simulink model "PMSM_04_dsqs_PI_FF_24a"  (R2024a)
settings: Solver=ode45  StartTime=0.0  StopTime=0.1  MaxStep=1e-4  RelTol=1e-3  AbsTol=1e-4  EnableMultiTasking=on
undefined symbols (not defined in the file): by, established, Flux, linkage, magnets, V
libraries: spsControlledVoltageSourceLib x3, spsCurrentMeasurementLib x3, slpidlib x2, spsPermanentMagnetSynchronousMachineLib x1, spspowerguiLib x1

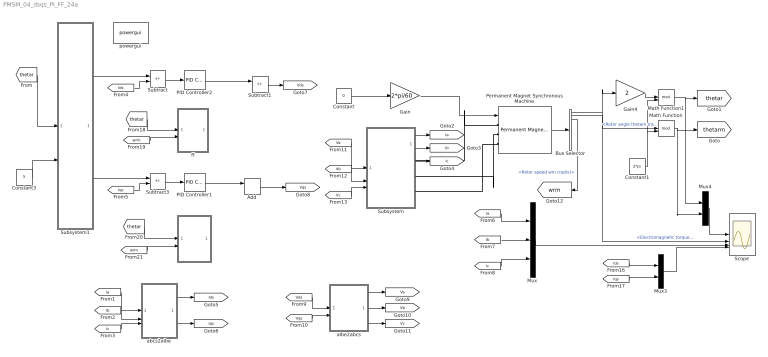
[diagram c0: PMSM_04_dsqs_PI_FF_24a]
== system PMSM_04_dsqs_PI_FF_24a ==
  Add : Sum
  Bus Selector : BusSelector  OutputSignals=Rotor angle thetam (rad),Electromagnetic torque Te (N*m),Rotor speed wm (rad/s)
  Constant : Constant  Value=0
  Constant1 : Constant  Value=2*pi
  Constant3 : Constant  Value=3
  FF : Subsystem
  Gain : Gain  Gain=2*pi/60
  Gain4 : Gain  Gain=2
  Math Function : Math  Operator=mod  SignedPower=on
  Math Function1 : Math  Operator=mod  SignedPower=on
  Mux : Mux  Inputs=3
  Mux3 : Mux  Inputs=2
  Mux4 : Mux  Inputs=2
  PID Controller1 : slpidlib/PID Controller  Controller=PI  Form=Parallel  TimeDomain=Continuous-time  UseExternalTs=off  SampleTime=1  IntegratorMethod=Forward Euler  FilterMethod=Forward Euler  ControllerParametersSource=internal  P=2*pi*500*0.00476  I=2*pi*500*0.423  UseKiTs=off  D=0  UseExternalDerivativeSource=off  N=100  UseFilter=on  TunerSelectOption=Transfer Function Based (PID Tuner App)  InitialConditionSource=internal  InitialConditionForIntegrator=0  InitialConditionForFilter=0  DifferentiatorICPrevScaledInput=0  ExternalReset=none  TrackingMode=off  Kt=1  LimitOutput=off  SatLimitsSource=internal  UpperSaturationLimit=inf  LowerSaturationLimit=-inf  LinearizeAsGain=on  AntiWindupMode=none  Kb=1  LimitIntegrator=off  UpperIntegratorSaturationLimit=inf  LowerIntegratorSaturationLimit=-inf  POutMin=[]  POutMax=[]  IOutMin=[]  IOutMax=[]  DOutMin=[]  DOutMax=[]  NOutMin=[]  NOutMax=[]  SumOutMin=[]  SumOutMax=[]  SaturationOutMin=[]  SaturationOutMax=[]  PParamMin=[]  PParamMax=[]  IParamMin=[]  IParamMax=[]  DParamMin=[]  DParamMax=[]  NParamMin=[]  NParamMax=[]  KbParamMin=[]  KbParamMax=[]  KtParamMin=[]  KtParamMax=[]  KbOutMin=[]  KbOutMax=[]  KtOutMin=[]  KtOutMax=[]  IntegratorOutMin=[]  IntegratorOutMax=[]  FilterOutMin=[]  FilterOutMax=[]  SumI1OutMin=[]  SumI1OutMax=[]  SumI2OutMin=[]  SumI2OutMax=[]  SumI3OutMin=[]  SumI3OutMax=[]  SumI4OutMin=[]  SumI4OutMax=[]  SumDOutMin=[]  SumDOutMax=[]  DifferentiatorOutMin=[]  DifferentiatorOutMax=[]  FilterDiffOutCoefMin=[]  FilterDiffOutCoefMax=[]  ReciprocalOutMin=[]  ReciprocalOutMax=[]  SumDenOutMin=[]  SumDenOutMax=[]  SumNumOutMin=[]  SumNumOutMax=[]  DivideOutMin=[]  DivideOutMax=[]  UdiffTsProdOutMin=[]  UdiffTsProdOutMax=[]  NTsProdOutMin=[]  NTsProdOutMax=[]  UintegralTsProdOutMin=[]  UintegralTsProdOutMax=[]  UngainTsProdOutMin=[]  UngainTsProdOutMax=[]  ClampingZeroOutDataTypeStr=Inherit: Inherit via back propagation  ClampingZeroOutMin=[]  ClampingZeroOutMax=[]  FilterDenConstantOutDataTypeStr=Inherit: Inherit via back propagation  FilterDenConstantOutMin=[]  FilterDenConstantOutMax=[]  PCopyOutDataTypeStr=Inherit: Inherit via back propagation  PCopyOutMin=[]  PCopyOutMax=[]  NCopyOutDataTypeStr=Inherit: Inherit via back propagation  NCopyOutMin=[]  NCopyOutMax=[]  IntegratorContinuousStateAttributes=''  IntegratorStateMustResolveToSignalObject=off  IntegratorRTWStateStorageClass=Auto  FilterContinuousStateAttributes=''  FilterStateMustResolveToSignalObject=off  FilterRTWStateStorageClass=Auto  ParallelPVariant=InternalParameters  IdealPVariant=Disabled  IVariant=InternalParameters  DVariant=Disabled  IntegratorVariant=Continuous  SatVariant=Disabled  AWVariant=Passthrough  PCopyVariant=Disabled  TRVariant=Disabled  FdbkBlocksVariant=Forward  IdealPFdbkVariant=Disabled  SatFdbkVariant=Disabled  DerivativeFilterVariant=Disabled  NVariant=Disabled  NCopyVariant=Disabled_SignalSpec  FilterICVariant=Disabled  IntegratorICVariant=InternalICs  ExternalResetVariant=Disabled  TRSumVariant=Passthrough  SumFdbkVariant=Disabled  SumVariant=Sum_PI  TsampFilterVariant=InternalTs  TsampNgainVariant=Passthrough  TsampIntegralVariant=Disabled_SignalSpec  ExternalSaturationOutDataTypeStr=Inherit: Same as second input  DerivativeSourceVariant=Disabled
  PID Controller2 : slpidlib/PID Controller  Controller=PI  Form=Parallel  TimeDomain=Continuous-time  UseExternalTs=off  SampleTime=1  IntegratorMethod=Forward Euler  FilterMethod=Forward Euler  ControllerParametersSource=internal  P=2*pi*500*0.00476  I=2*pi*500*0.423  UseKiTs=off  D=0  UseExternalDerivativeSource=off  N=100  UseFilter=on  TunerSelectOption=Transfer Function Based (PID Tuner App)  InitialConditionSource=internal  InitialConditionForIntegrator=0  InitialConditionForFilter=0  DifferentiatorICPrevScaledInput=0  ExternalReset=none  TrackingMode=off  Kt=1  LimitOutput=off  SatLimitsSource=internal  UpperSaturationLimit=inf  LowerSaturationLimit=-inf  LinearizeAsGain=on  AntiWindupMode=none  Kb=1  LimitIntegrator=off  UpperIntegratorSaturationLimit=inf  LowerIntegratorSaturationLimit=-inf  POutMin=[]  POutMax=[]  IOutMin=[]  IOutMax=[]  DOutMin=[]  DOutMax=[]  NOutMin=[]  NOutMax=[]  SumOutMin=[]  SumOutMax=[]  SaturationOutMin=[]  SaturationOutMax=[]  PParamMin=[]  PParamMax=[]  IParamMin=[]  IParamMax=[]  DParamMin=[]  DParamMax=[]  NParamMin=[]  NParamMax=[]  KbParamMin=[]  KbParamMax=[]  KtParamMin=[]  KtParamMax=[]  KbOutMin=[]  KbOutMax=[]  KtOutMin=[]  KtOutMax=[]  IntegratorOutMin=[]  IntegratorOutMax=[]  FilterOutMin=[]  FilterOutMax=[]  SumI1OutMin=[]  SumI1OutMax=[]  SumI2OutMin=[]  SumI2OutMax=[]  SumI3OutMin=[]  SumI3OutMax=[]  SumI4OutMin=[]  SumI4OutMax=[]  SumDOutMin=[]  SumDOutMax=[]  DifferentiatorOutMin=[]  DifferentiatorOutMax=[]  FilterDiffOutCoefMin=[]  FilterDiffOutCoefMax=[]  ReciprocalOutMin=[]  ReciprocalOutMax=[]  SumDenOutMin=[]  SumDenOutMax=[]  SumNumOutMin=[]  SumNumOutMax=[]  DivideOutMin=[]  DivideOutMax=[]  UdiffTsProdOutMin=[]  UdiffTsProdOutMax=[]  NTsProdOutMin=[]  NTsProdOutMax=[]  UintegralTsProdOutMin=[]  UintegralTsProdOutMax=[]  UngainTsProdOutMin=[]  UngainTsProdOutMax=[]  ClampingZeroOutDataTypeStr=Inherit: Inherit via back propagation  ClampingZeroOutMin=[]  ClampingZeroOutMax=[]  FilterDenConstantOutDataTypeStr=Inherit: Inherit via back propagation  FilterDenConstantOutMin=[]  FilterDenConstantOutMax=[]  PCopyOutDataTypeStr=Inherit: Inherit via back propagation  PCopyOutMin=[]  PCopyOutMax=[]  NCopyOutDataTypeStr=Inherit: Inherit via back propagation  NCopyOutMin=[]  NCopyOutMax=[]  IntegratorContinuousStateAttributes=''  IntegratorStateMustResolveToSignalObject=off  IntegratorRTWStateStorageClass=Auto  FilterContinuousStateAttributes=''  FilterStateMustResolveToSignalObject=off  FilterRTWStateStorageClass=Auto  ParallelPVariant=InternalParameters  IdealPVariant=Disabled  IVariant=InternalParameters  DVariant=Disabled  IntegratorVariant=Continuous  SatVariant=Disabled  AWVariant=Passthrough  PCopyVariant=Disabled  TRVariant=Disabled  FdbkBlocksVariant=Forward  IdealPFdbkVariant=Disabled  SatFdbkVariant=Disabled  DerivativeFilterVariant=Disabled  NVariant=Disabled  NCopyVariant=Disabled_SignalSpec  FilterICVariant=Disabled  IntegratorICVariant=InternalICs  ExternalResetVariant=Disabled  TRSumVariant=Passthrough  SumFdbkVariant=Disabled  SumVariant=Sum_PI  TsampFilterVariant=InternalTs  TsampNgainVariant=Passthrough  TsampIntegralVariant=Disabled_SignalSpec  ExternalSaturationOutDataTypeStr=Inherit: Same as second input  DerivativeSourceVariant=Disabled
  Permanent Magnet Synchronous Machine : spsPermanentMagnetSynchronousMachineLib/Permanent Magnet Synchronous Machine  NbPhases=3  FluxDistribution=Sinusoidal  RotorType=Round  MechanicalLoad=Speed w  PresetModel=No  ShowDetailedParameters=on  MeasurementBus=off  Resistance=0.423  Inductance=8.5e-3  dqInductances=[8.5e-3,8.5e-3]  La=0.00476  MachineConstant=Flux linkage established by magnets (V.s)  Flux=0.422  VoltageCst=153.0847  TorqueCst=1.266  Flat=120  Mechanical=[0.03 0.04 4 0]  PolePairs=2  InitialConditions=[0,0, 0,0]  InitialConditions5ph=[0 0 0 0 0 0]  RefAngle=Aligned with phase A axis (original Park)  IterativeDiscreteModel=Trapezoidal non iterative  TsBlock=-1  TsPowergui=0
  Scope : Scope  NumInputPorts=4
  Subsystem : Subsystem
  Subsystem1 : Subsystem
  Subtract : Sum  Inputs=+-
  Subtract1 : Sum  Inputs=+-
  Subtract3 : Sum  Inputs=+-
  abcs2albe : Subsystem
  albe2abcs : Subsystem
  ff : Subsystem
  powergui : spspowerguiLib/powergui  Priority=1  SimulationMode=Continuous  SampleTime=50e-6  frequency=60  Iterations=50  frequencyindice=0  Pbase=100e6  ErrMax=1e-4  UnitsV=kV  UnitsW=MW  buscounter=0  FunctionMessages=off  echomessages=off  EnableUseOfTLC=off  CurrentSourceSwitches=off  DisableSnubberDevices=on  DisableRonSwitches=on  DisableVfSwitches=on  DisplayEquations=off  AutomaticDiscreteSolvers=off  SolverType=Tustin  Interpol=off  ExternalGateDelay=off  methode=off  Ts=0  x0status=blocks  SPID=on  SwTol=0  HookPort=off  NonlinearTolerance=1e-4  nMaxIteration=100  ContinueOnMaxIteration=off  RestoreLinks=warning  ResistiveCurrentMeasurement=off  Frange=[0:2:500]  Ylog=off  Xlog=on  ShowGrid=off  save=off  variable=ZData  structure=0  ZoomFFT=off  StartTime=0.0  cycles=1  DisplayStyle=1  fundamental=60  FreqAxis=off  MaxFrequency=1000  frequencyindicesteady=1  RmsSteady=1  display=off
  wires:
  Gain/1 -> Permanent Magnet Synchronous Machine/1
  Constant/1 -> Gain/1
  Subtract/1 -> PID Controller2/1
  Permanent Magnet Synchronous Machine/1 -> Bus Selector/1
  Mux/1 -> Scope/3
  Bus Selector/2 -> Scope/2  "<Electromagnetic torque Te (N*m)>"
  Bus Selector/1 -> Gain4/1, Math Function/1  "<Rotor angle thetam (rad)>"
  Constant1/1 -> Math Function1/2, Math Function/2
  Math Function/1 -> Mux4/2, [thetarm]
  Gain4/1 -> Math Function1/1
  Math Function1/1 -> Mux4/1, [thetar]
  [thetar] -> Subsystem1/1(In1)
  Constant3/1 -> Subsystem1/2(In2)
  Subtract3/1 -> PID Controller1/1
  Subsystem1/1(Out1) -> Subtract/1
  Subsystem1/2(Out2) -> Subtract3/1
  Subsystem/1(Out1) -> [Ia]
  Subsystem/2(Out2) -> [Ib]
  Subsystem/3(Out3) -> [Ic]
  [Ids] -> Subtract/2
  [Iqs] -> Subtract3/2
  [Ia] -> Mux/1
  [Ib] -> Mux/2
  [Ic] -> Mux/3
  Mux3/1 -> Scope/4
  [Ids] -> Mux3/1
  [Iqs] -> Mux3/2
  Mux4/1 -> Scope/1
  [Vds] -> albe2abcs/1(alpha)
  [Vqs] -> albe2abcs/2(beta)
  albe2abcs/1(as) -> [Va]
  albe2abcs/2(bs) -> [Vb]
  albe2abcs/3(cs) -> [Vc]
  [Ia] -> abcs2albe/1(as)
  [Ib] -> abcs2albe/2(bs)
  [Ic] -> abcs2albe/3(cs)
  abcs2albe/1(alpha) -> [Ids]
  abcs2albe/2(beta) -> [Iqs]
  [Vc] -> Subsystem/3(In3)
  [Vb] -> Subsystem/2(In2)
  [Va] -> Subsystem/1(In1)
  PID Controller2/1 -> Subtract1/1
  Subtract1/1 -> [Vds]
  PID Controller1/1 -> Add/1
  Add/1 -> [Vqs]
  Bus Selector/3 -> [wrm]  "<Rotor speed wm (rad/s)>"
  [thetar] -> ff/1(In1)
  [wrm] -> ff/2(In2)
  [thetar] -> FF/1(In1)
  [wrm] -> FF/2(In2)
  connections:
  Subsystem/RConn1 -- Permanent Magnet Synchronous Machine/LConn1
  Permanent Magnet Synchronous Machine/LConn2 -- Subsystem/RConn2
  Subsystem/RConn3 -- Permanent Magnet Synchronous Machine/LConn3

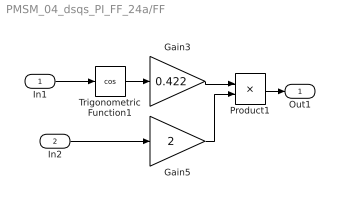
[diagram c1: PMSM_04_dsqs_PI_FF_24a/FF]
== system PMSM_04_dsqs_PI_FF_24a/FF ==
  In1 : Inport
  In2 : Inport  Port=2
  Gain3 : Gain  Gain=0.422
  Gain5 : Gain  Gain=2
  Product1 : Product
  Trigonometric Function1 : Trigonometry  Operator=cos
  Out1 : Outport
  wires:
  Product1/1 -> Out1/1
  Gain3/1 -> Product1/1
  In2/1 -> Gain5/1
  In1/1 -> Trigonometric Function1/1
  Trigonometric Function1/1 -> Gain3/1
  Gain5/1 -> Product1/2

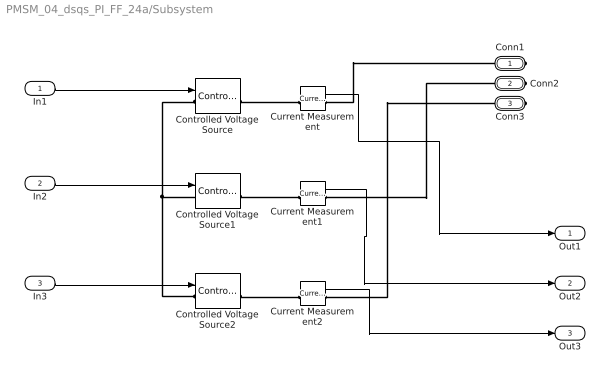
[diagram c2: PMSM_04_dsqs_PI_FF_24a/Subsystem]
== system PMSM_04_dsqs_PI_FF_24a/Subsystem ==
  In1 : Inport
  In2 : Inport  Port=2
  In3 : Inport  Port=3
  Controlled Voltage Source : spsControlledVoltageSourceLib/Controlled Voltage Source  Initialize=on  Source_Type=AC  Amplitude=0  Phase=0  Frequency=0  Measurements=None
  Controlled Voltage Source1 : spsControlledVoltageSourceLib/Controlled Voltage Source  Initialize=on  Source_Type=AC  Amplitude=0  Phase=0  Frequency=0  Measurements=None
  Controlled Voltage Source2 : spsControlledVoltageSourceLib/Controlled Voltage Source  Initialize=on  Source_Type=AC  Amplitude=0  Phase=0  Frequency=0  Measurements=None
  Current Measurement : spsCurrentMeasurementLib/Current Measurement  PhasorSimulation=off  OutputType=Complex  PSBequivalent=0
  Current Measurement1 : spsCurrentMeasurementLib/Current Measurement  PhasorSimulation=off  OutputType=Complex  PSBequivalent=0
  Current Measurement2 : spsCurrentMeasurementLib/Current Measurement  PhasorSimulation=off  OutputType=Complex  PSBequivalent=0
  Conn1 : PMIOPort  Side=Right
  Conn2 : PMIOPort  Port=2  Side=Right
  Conn3 : PMIOPort  Port=3  Side=Right
  Out1 : Outport
  Out2 : Outport  Port=2
  Out3 : Outport  Port=3
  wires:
  Current Measurement1/1 -> Out2/1
  In3/1 -> Controlled Voltage Source2/1
  In2/1 -> Controlled Voltage Source1/1
  In1/1 -> Controlled Voltage Source/1
  Current Measurement2/1 -> Out3/1
  Current Measurement/1 -> Out1/1
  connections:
  Current Measurement/RConn1 -- Conn1/RConn1
  Controlled Voltage Source/LConn1 -- Controlled Voltage Source1/LConn1 -- Controlled Voltage Source2/LConn1
  Controlled Voltage Source/RConn1 -- Current Measurement/LConn1
  Conn2/RConn1 -- Current Measurement1/RConn1
  Current Measurement2/RConn1 -- Conn3/RConn1
  Controlled Voltage Source1/RConn1 -- Current Measurement1/LConn1
  Controlled Voltage Source2/RConn1 -- Current Measurement2/LConn1

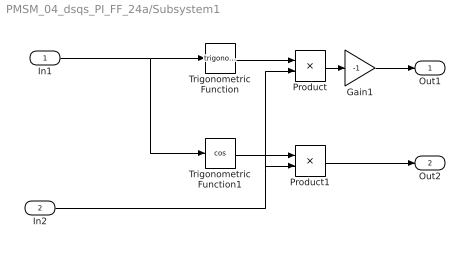
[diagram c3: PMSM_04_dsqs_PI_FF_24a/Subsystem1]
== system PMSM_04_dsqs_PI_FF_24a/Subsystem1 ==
  In1 : Inport
  In2 : Inport  Port=2
  Gain1 : Gain  Gain=-1
  Product : Product
  Product1 : Product
  Trigonometric Function : Trigonometry
  Trigonometric Function1 : Trigonometry  Operator=cos
  Out1 : Outport
  Out2 : Outport  Port=2
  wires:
  Trigonometric Function1/1 -> Product1/1
  Product/1 -> Gain1/1
  Product1/1 -> Out2/1
  In1/1 -> Trigonometric Function1/1, Trigonometric Function/1
  Trigonometric Function/1 -> Product/1
  Gain1/1 -> Out1/1
  In2/1 -> Product/2, Product1/2

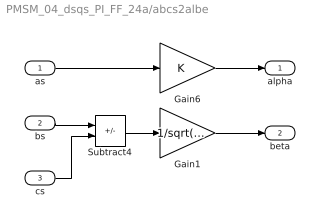
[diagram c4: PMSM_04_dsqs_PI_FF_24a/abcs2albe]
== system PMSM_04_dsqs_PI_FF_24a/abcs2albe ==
  as : Inport
  bs : Inport  Port=2
  cs : Inport  Port=3
  Gain1 : Gain  Gain=1/sqrt(3)
  Gain6 : Gain
  Subtract4 : Sum  Inputs=+-
  alpha : Outport
  beta : Outport  Port=2
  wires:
  bs/1 -> Subtract4/1
  as/1 -> Gain6/1
  cs/1 -> Subtract4/2
  Gain1/1 -> beta/1
  Subtract4/1 -> Gain1/1
  Gain6/1 -> alpha/1

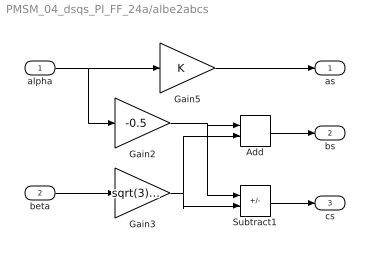
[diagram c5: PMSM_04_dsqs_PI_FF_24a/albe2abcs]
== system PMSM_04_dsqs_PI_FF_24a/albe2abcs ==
  alpha : Inport
  beta : Inport  Port=2
  Add : Sum
  Gain2 : Gain  Gain=-0.5
  Gain3 : Gain  Gain=sqrt(3)/2
  Gain5 : Gain
  Subtract1 : Sum  Inputs=+-
  as : Outport
  bs : Outport  Port=2
  cs : Outport  Port=3
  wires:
  alpha/1 -> Gain2/1, Gain5/1
  Gain3/1 -> Subtract1/2, Add/2
  Gain2/1 -> Subtract1/1, Add/1
  Add/1 -> bs/1
  Subtract1/1 -> cs/1
  beta/1 -> Gain3/1
  Gain5/1 -> as/1

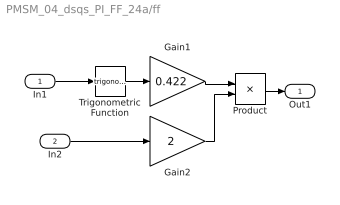
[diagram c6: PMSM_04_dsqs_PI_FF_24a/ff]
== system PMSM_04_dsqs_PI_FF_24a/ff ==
  In1 : Inport
  In2 : Inport  Port=2
  Gain1 : Gain  Gain=0.422
  Gain2 : Gain  Gain=2
  Product : Product
  Trigonometric Function : Trigonometry
  Out1 : Outport
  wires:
  Trigonometric Function/1 -> Gain1/1
  In1/1 -> Trigonometric Function/1
  Product/1 -> Out1/1
  Gain1/1 -> Product/1
  In2/1 -> Gain2/1
  Gain2/1 -> Product/2
